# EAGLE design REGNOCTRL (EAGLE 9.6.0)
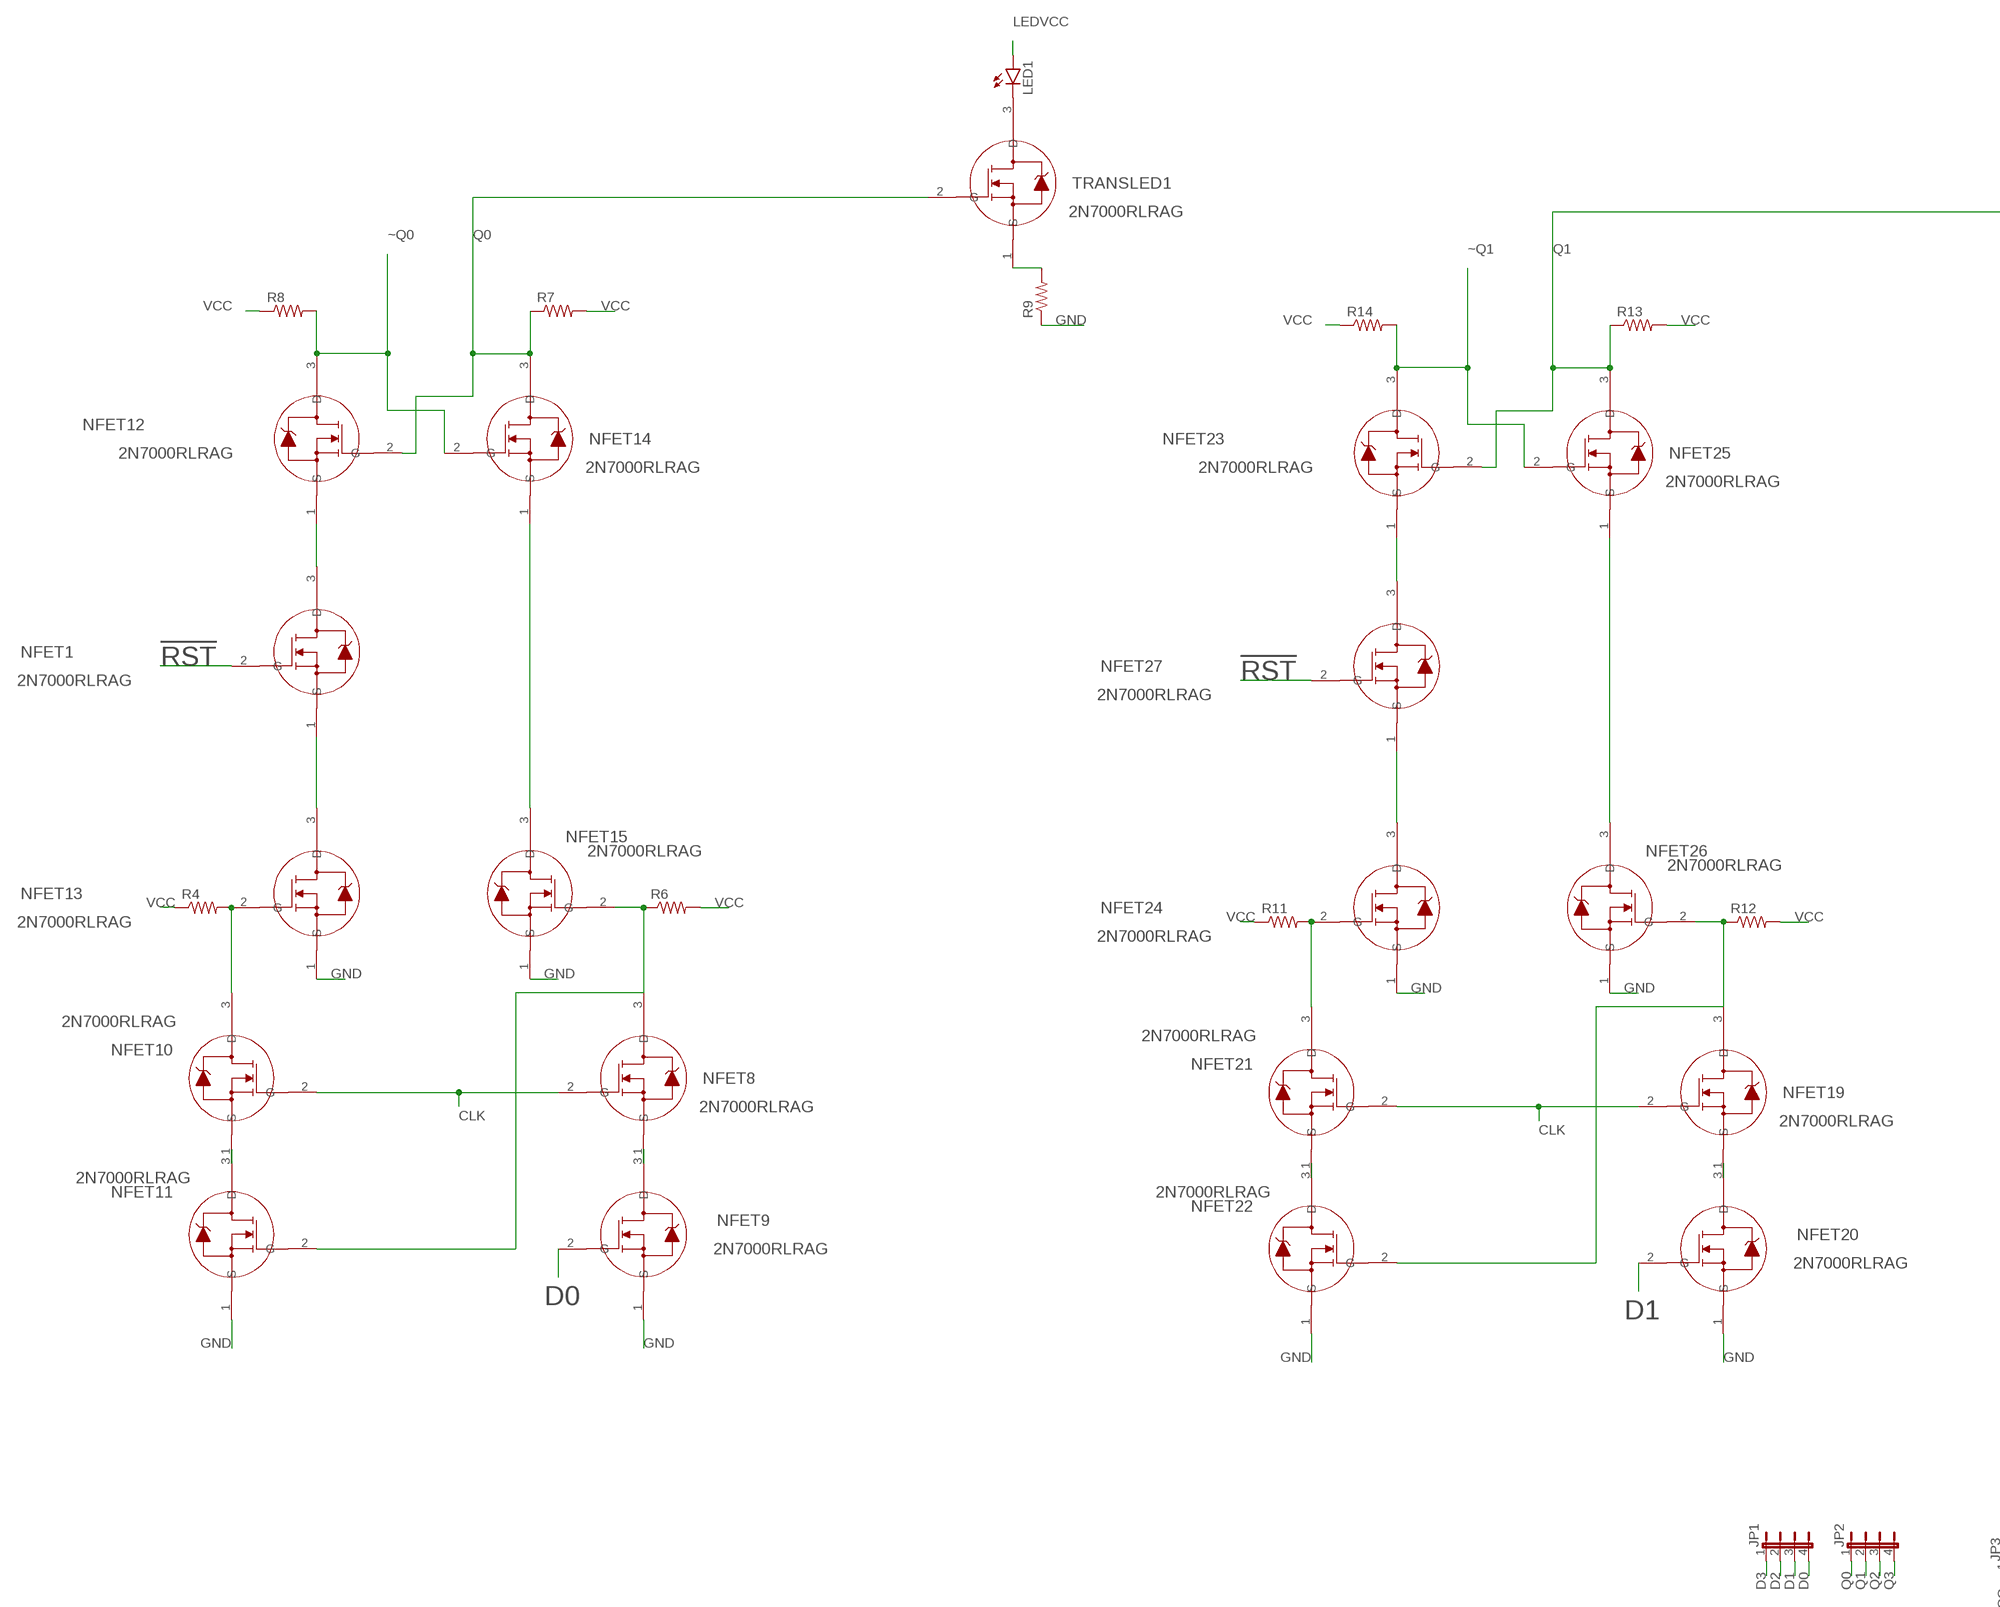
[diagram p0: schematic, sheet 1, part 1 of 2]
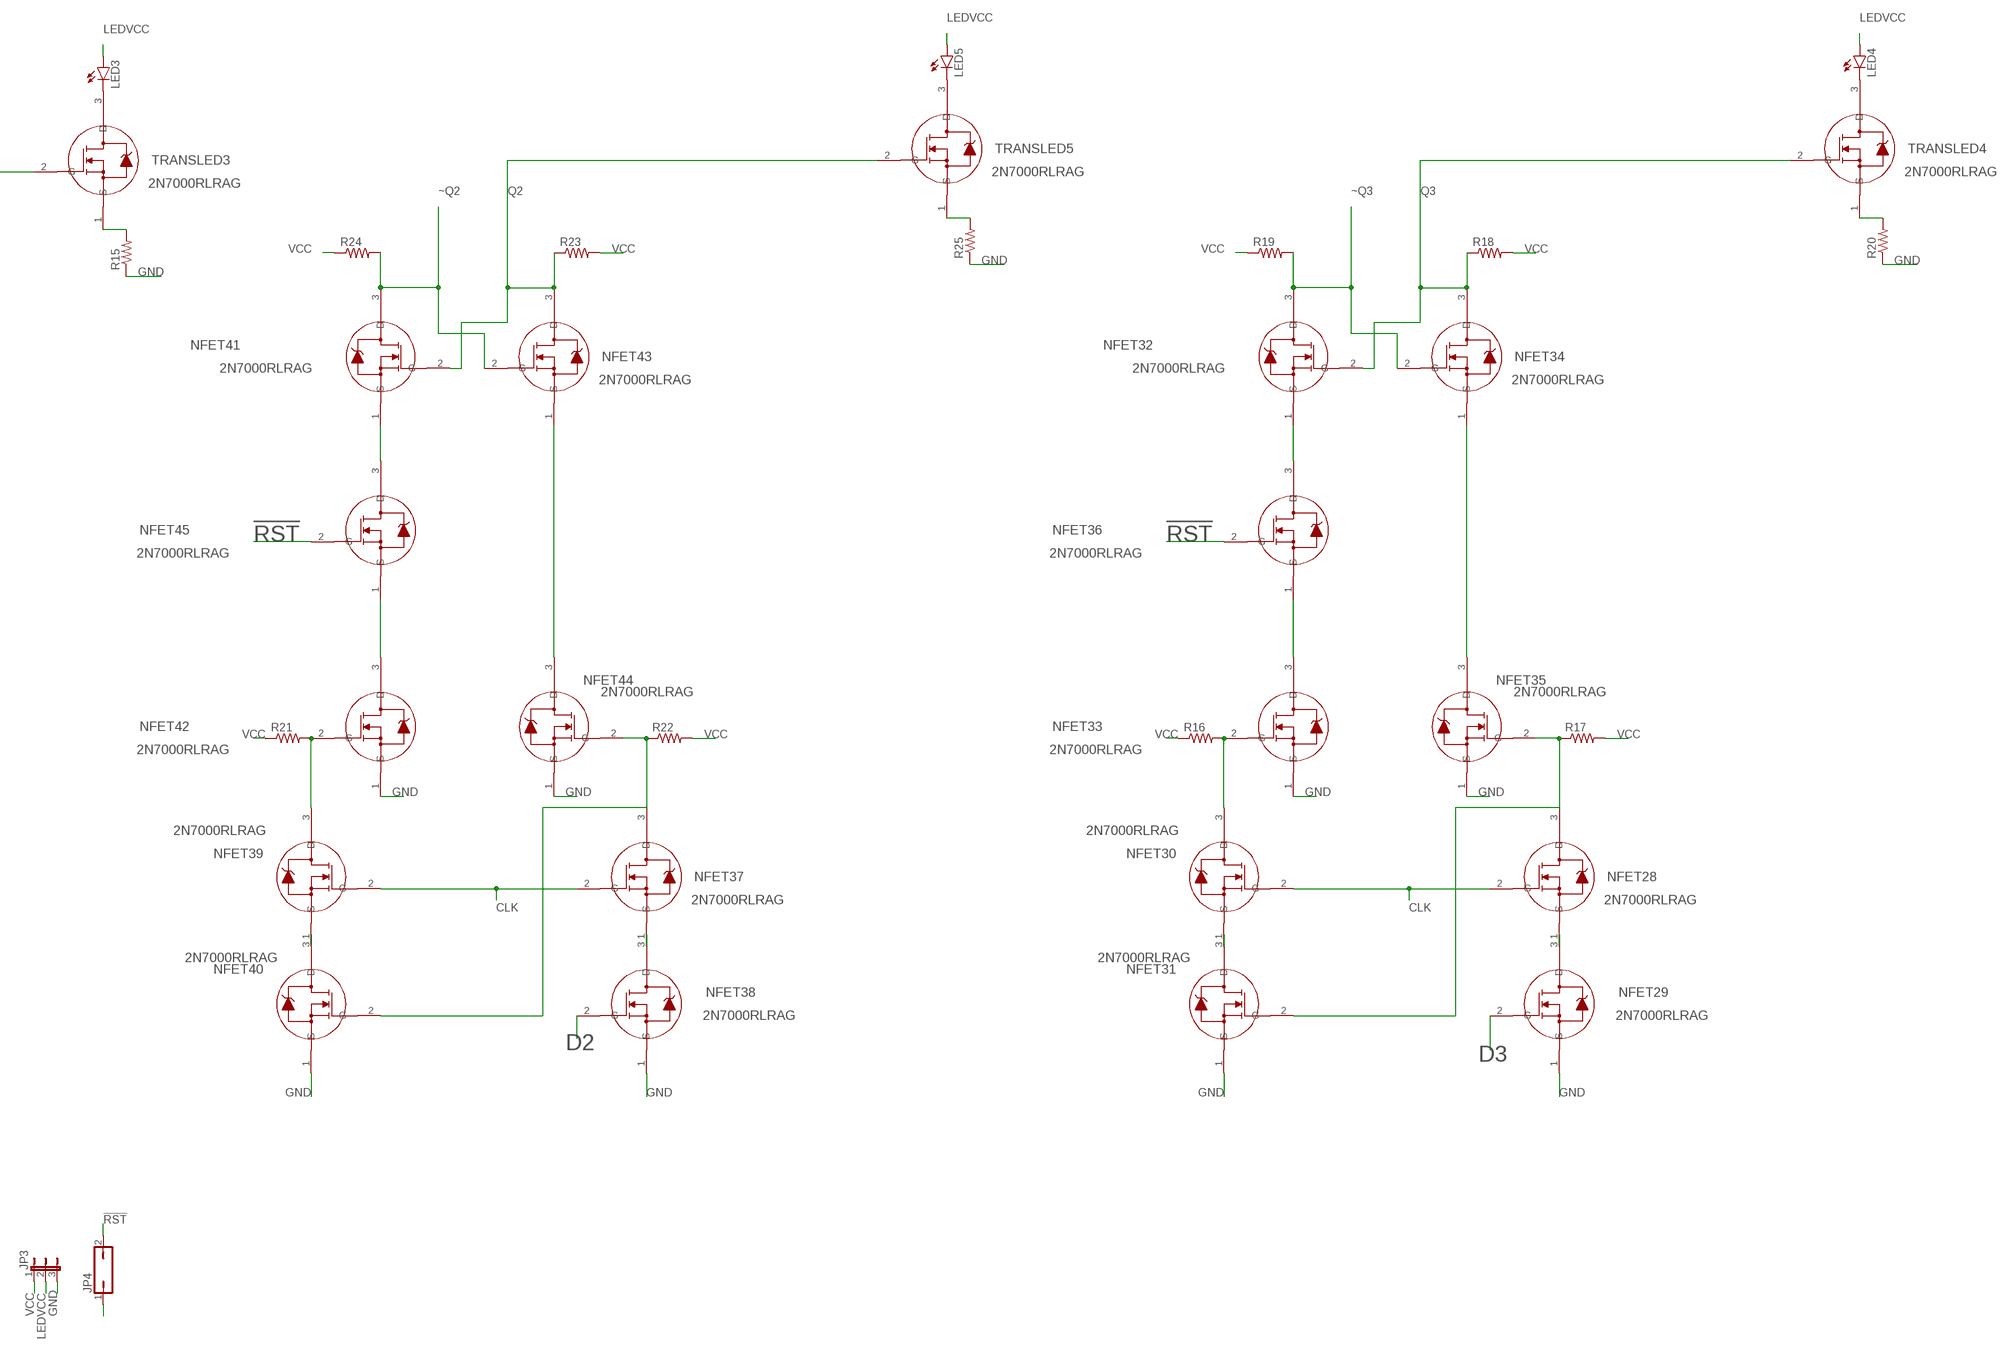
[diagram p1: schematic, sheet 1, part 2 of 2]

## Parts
JP1  JP4E  [JP4]
JP2  JP4E  [JP4]
JP3  JP2E  [JP2]
JP4  JP1Q  [JP1]
LED1  LED3MM  [LED3MM]
LED3  LED3MM  [LED3MM]
LED4  LED3MM  [LED3MM]
LED5  LED3MM  [LED3MM]
NFET1  2N7000RLRAG  [TO-92_ONS]
NFET8  2N7000RLRAG  [TO-92_ONS]
NFET9  2N7000RLRAG  [TO-92_ONS]
NFET10  2N7000RLRAG  [TO-92_ONS]
NFET11  2N7000RLRAG  [TO-92_ONS]
NFET12  2N7000RLRAG  [TO-92_ONS]
NFET13  2N7000RLRAG  [TO-92_ONS]
NFET14  2N7000RLRAG  [TO-92_ONS]
NFET15  2N7000RLRAG  [TO-92_ONS]
NFET19  2N7000RLRAG  [TO-92_ONS]
NFET20  2N7000RLRAG  [TO-92_ONS]
NFET21  2N7000RLRAG  [TO-92_ONS]
NFET22  2N7000RLRAG  [TO-92_ONS]
NFET23  2N7000RLRAG  [TO-92_ONS]
NFET24  2N7000RLRAG  [TO-92_ONS]
NFET25  2N7000RLRAG  [TO-92_ONS]
NFET26  2N7000RLRAG  [TO-92_ONS]
NFET27  2N7000RLRAG  [TO-92_ONS]
NFET28  2N7000RLRAG  [TO-92_ONS]
NFET29  2N7000RLRAG  [TO-92_ONS]
NFET30  2N7000RLRAG  [TO-92_ONS]
NFET31  2N7000RLRAG  [TO-92_ONS]
NFET32  2N7000RLRAG  [TO-92_ONS]
NFET33  2N7000RLRAG  [TO-92_ONS]
NFET34  2N7000RLRAG  [TO-92_ONS]
NFET35  2N7000RLRAG  [TO-92_ONS]
NFET36  2N7000RLRAG  [TO-92_ONS]
NFET37  2N7000RLRAG  [TO-92_ONS]
NFET38  2N7000RLRAG  [TO-92_ONS]
NFET39  2N7000RLRAG  [TO-92_ONS]
NFET40  2N7000RLRAG  [TO-92_ONS]
NFET41  2N7000RLRAG  [TO-92_ONS]
NFET42  2N7000RLRAG  [TO-92_ONS]
NFET43  2N7000RLRAG  [TO-92_ONS]
NFET44  2N7000RLRAG  [TO-92_ONS]
NFET45  2N7000RLRAG  [TO-92_ONS]
R4  R-US_0204/7  [0204/7]
R6  R-US_0204/7  [0204/7]
R7  R-US_0204/7  [0204/7]
R8  R-US_0204/7  [0204/7]
R9  R-US_0204/7  [0204/7]
R11  R-US_0204/7  [0204/7]
R12  R-US_0204/7  [0204/7]
R13  R-US_0204/7  [0204/7]
R14  R-US_0204/7  [0204/7]
R15  R-US_0204/7  [0204/7]
R16  R-US_0204/7  [0204/7]
R17  R-US_0204/7  [0204/7]
R18  R-US_0204/7  [0204/7]
R19  R-US_0204/7  [0204/7]
R20  R-US_0204/7  [0204/7]
R21  R-US_0204/7  [0204/7]
R22  R-US_0204/7  [0204/7]
R23  R-US_0204/7  [0204/7]
R24  R-US_0204/7  [0204/7]
R25  R-US_0204/7  [0204/7]
TRANSLED1  2N7000RLRAG  [TO-92_ONS]
TRANSLED3  2N7000RLRAG  [TO-92_ONS]
TRANSLED4  2N7000RLRAG  [TO-92_ONS]
TRANSLED5  2N7000RLRAG  [TO-92_ONS]

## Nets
!RST: JP4.2 NFET1.2(G) NFET27.2(G) NFET36.2(G) NFET45.2(G)
CLK: JP4.1 NFET8.2(G) NFET10.2(G) NFET19.2(G) NFET21.2(G) NFET28.2(G) NFET30.2(G) NFET37.2(G) NFET39.2(G)
D0: JP1.4 NFET9.2(G)
D1: JP1.3 NFET20.2(G)
D2: JP1.2 NFET38.2(G)
D3: JP1.1 NFET29.2(G)
GND: JP3.3 NFET9.1(S) NFET11.1(S) NFET13.1(S) NFET15.1(S) NFET20.1(S) NFET22.1(S) NFET24.1(S) NFET26.1(S) NFET29.1(S) NFET31.1(S) NFET33.1(S) NFET35.1(S) NFET38.1(S) NFET40.1(S) NFET42.1(S) NFET44.1(S) R9.1 R15.1 R20.1 R25.1
LEDVCC: JP3.2 LED1.A LED3.A LED4.A LED5.A
N$1: NFET8.1(S) NFET9.3(D)
N$2: NFET1.3(D) NFET12.1(S)
N$3: NFET10.1(S) NFET11.3(D)
N$4: NFET10.3(D) NFET13.2(G) R4.2
N$5: NFET1.1(S) NFET13.3(D)
N$6: NFET14.1(S) NFET15.3(D)
N$7: NFET8.3(D) NFET11.2(G) NFET15.2(G) R6.1
N$8: LED1.K(C) TRANSLED1.3(D)
N$10: R9.2 TRANSLED1.1(S)
N$19: NFET19.1(S) NFET20.3(D)
N$20: NFET21.1(S) NFET22.3(D)
N$21: NFET21.3(D) NFET24.2(G) R11.2
N$22: NFET25.1(S) NFET26.3(D)
N$23: NFET19.3(D) NFET22.2(G) NFET26.2(G) R12.1
N$24: LED3.K(C) TRANSLED3.3(D)
N$25: R15.2 TRANSLED3.1(S)
N$26: NFET23.1(S) NFET27.3(D)
N$27: NFET24.3(D) NFET27.1(S)
N$28: NFET28.1(S) NFET29.3(D)
N$29: NFET30.1(S) NFET31.3(D)
N$30: NFET30.3(D) NFET33.2(G) R16.2
N$31: NFET34.1(S) NFET35.3(D)
N$32: NFET28.3(D) NFET31.2(G) NFET35.2(G) R17.1
N$33: LED4.K(C) TRANSLED4.3(D)
N$34: R20.2 TRANSLED4.1(S)
N$35: NFET32.1(S) NFET36.3(D)
N$36: NFET33.3(D) NFET36.1(S)
N$37: NFET37.1(S) NFET38.3(D)
N$38: NFET39.1(S) NFET40.3(D)
N$39: NFET39.3(D) NFET42.2(G) R21.2
N$40: NFET43.1(S) NFET44.3(D)
N$41: NFET37.3(D) NFET40.2(G) NFET44.2(G) R22.1
N$42: LED5.K(C) TRANSLED5.3(D)
N$43: R25.2 TRANSLED5.1(S)
N$44: NFET41.1(S) NFET45.3(D)
N$45: NFET42.3(D) NFET45.1(S)
Q0: JP2.1 NFET12.2(G) NFET14.3(D) R7.1 TRANSLED1.2(G)
Q1: JP2.2 NFET23.2(G) NFET25.3(D) R13.1 TRANSLED3.2(G)
Q2: JP2.3 NFET41.2(G) NFET43.3(D) R23.1 TRANSLED5.2(G)
Q3: JP2.4 NFET32.2(G) NFET34.3(D) R18.1 TRANSLED4.2(G)
VCC: JP3.1 R4.1 R6.2 R7.2 R8.1 R11.1 R12.2 R13.2 R14.1 R16.1 R17.2 R18.2 R19.1 R21.1 R22.2 R23.2 R24.1
~Q0: NFET12.3(D) NFET14.2(G) R8.2
~Q1: NFET23.3(D) NFET25.2(G) R14.2
~Q2: NFET41.3(D) NFET43.2(G) R24.2
~Q3: NFET32.3(D) NFET34.2(G) R19.2

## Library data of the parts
JP1 JP2 = jumper:JP4E: JUMPER
JP3 = jumper:JP2E: JUMPER
JP4 = jumper:JP1Q: JUMPER
LED1 LED3-LED5 = led:LED: LED
NFET1 NFET8-NFET15 NFET19-NFET45 TRANSLED1 TRANSLED3-TRANSLED5 = Transistor(MOSFET):2N7000RLRAG; COPYRIGHT: Copyright (C) 2022 Ultra Librarian. All rights reserved.; MANUFACTURER_PART_NUMBER: 2N7000RLRAG; MFR_NAME: onsemi
R4 R6-R9 R11-R25 = rcl:R-US_: RESISTOR, American symbol; SPICEPREFIX: R

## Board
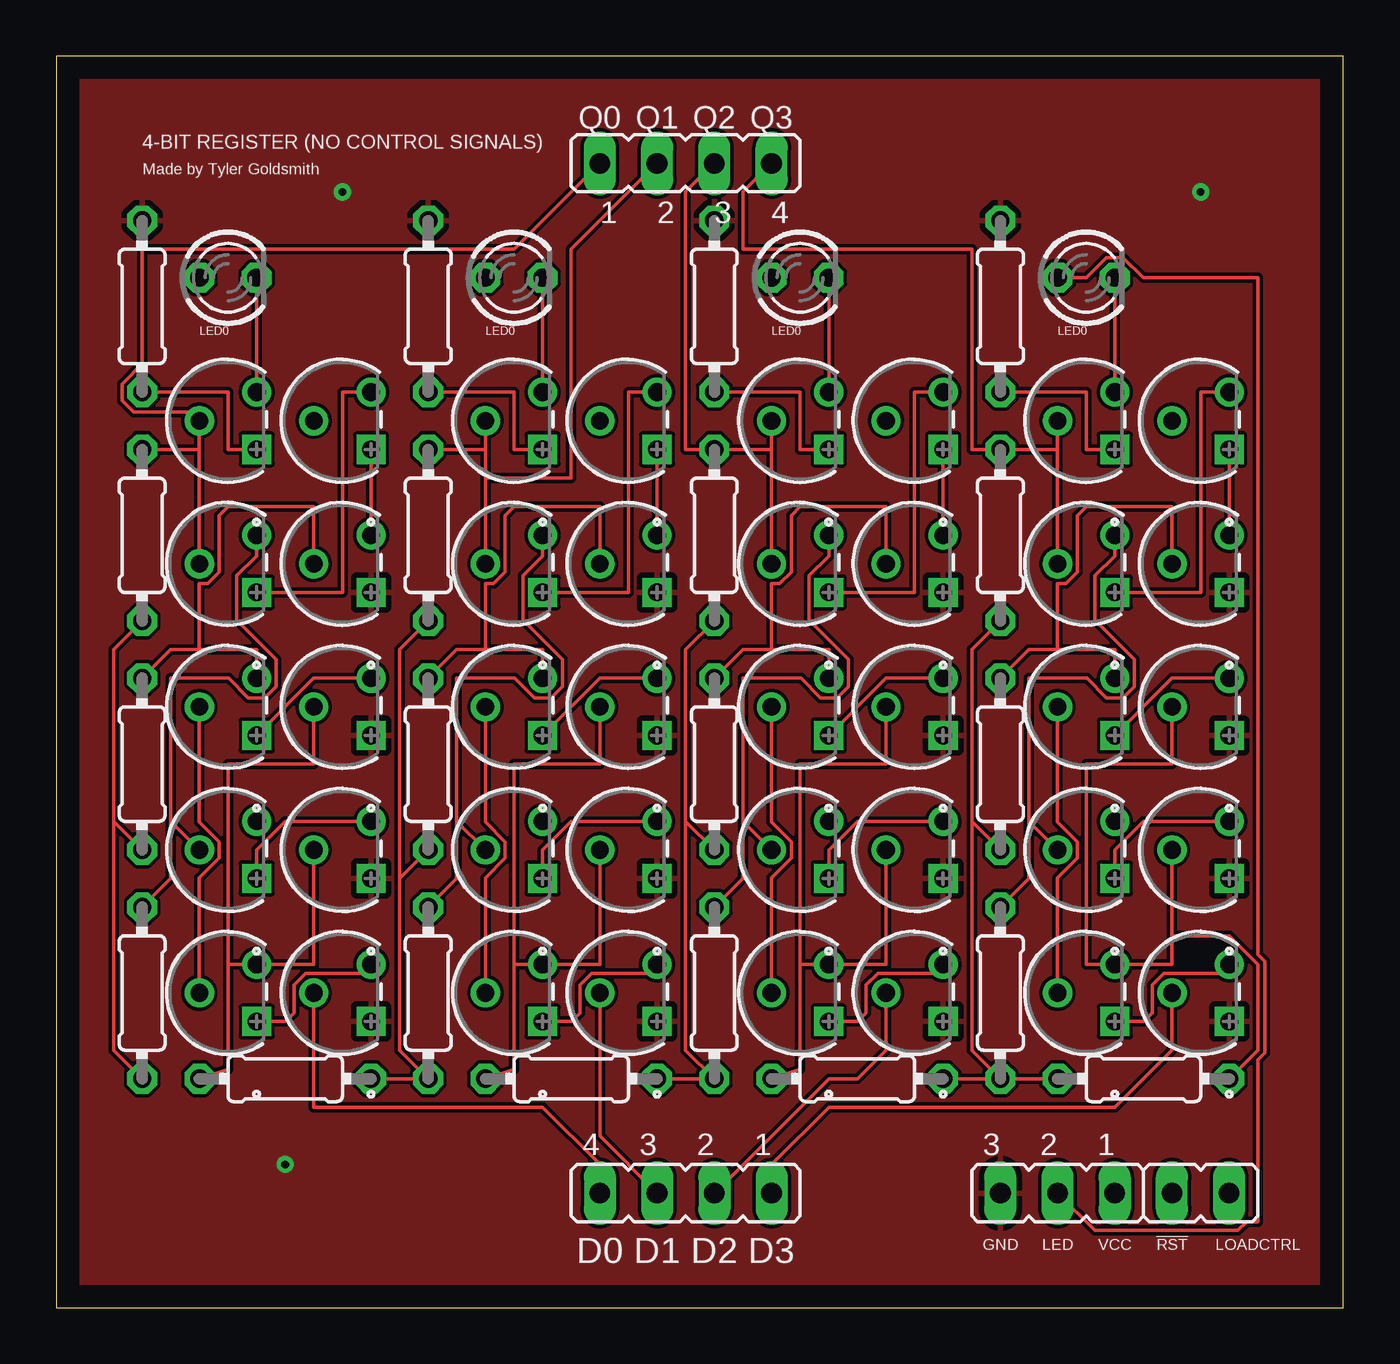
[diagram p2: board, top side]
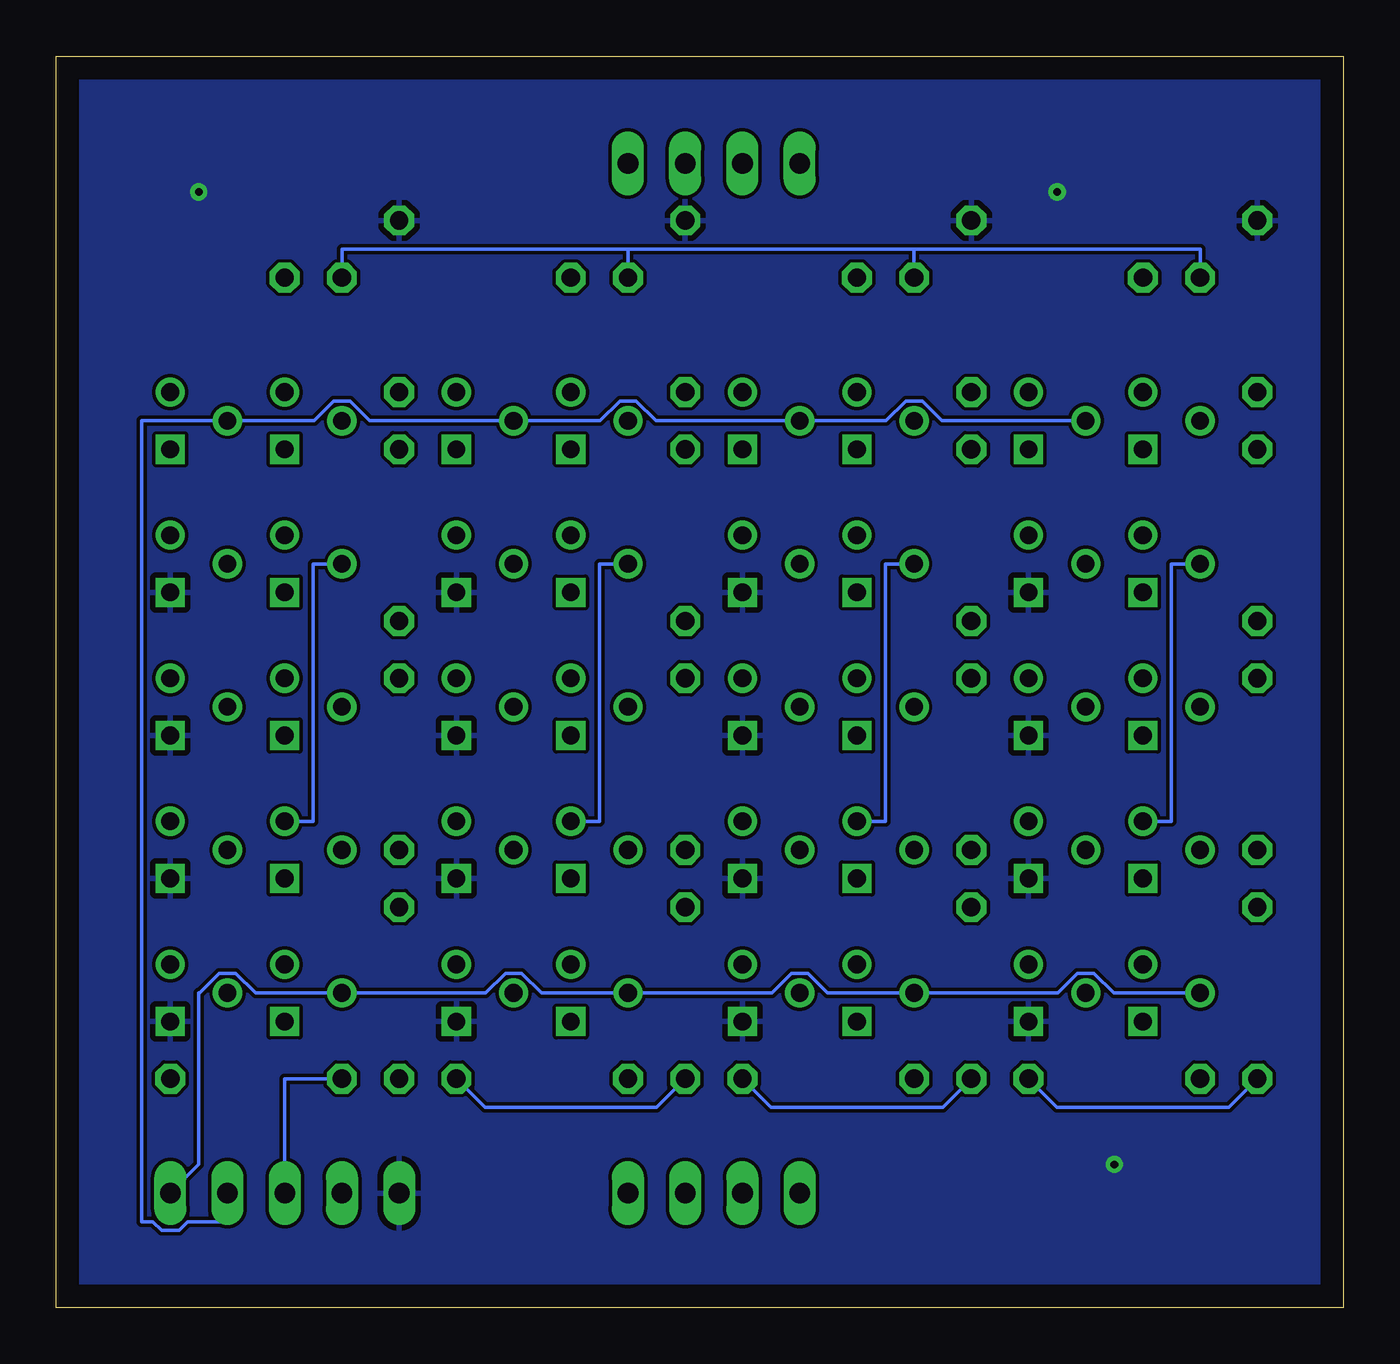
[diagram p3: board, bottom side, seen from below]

Size 57.13 x 55.55 mm. Coordinates in mm from the lower left corner, seen from the top.
Outline: 0,0 57.13,0 57.13,55.55 0,55.55 0,0
Copper layers (1*16): Top 0.035mm / dielectric 1.5mm / Bottom 0.035mm
Design rules "default": minimum track width 6mil, minimum drill 0.35mm, track to track 6mil, track to pad 6mil, pad to pad 6mil, via to via 6mil, smd to smd 6mil, copper to edge 40mil, drill to drill 6mil, minimum pad ring 10mil, minimum via ring 8mil, stop-mask expansion 4mil, vias tented up to drill 0mil, thermal gap 10mil

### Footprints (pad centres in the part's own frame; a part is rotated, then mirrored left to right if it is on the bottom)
JP4 = drill 0.914 long: 1 -3.81,0; 2 -1.27,0; 3 1.27,0; 4 3.81,0
JP2 = drill 0.914 long: 1 -2.54,0; 2 0,0; 3 2.54,0
JP1 = drill 0.914 long: 1 0,-1.27; 2 0,1.27
LED3MM = drill 0.813 octagon: A -1.27,0; K 1.27,0
TO-92_ONS = drill 0.787 pad 1.295 square: 1 0,0 | drill 0.787 pad 1.295: 2 1.27,2.54; 3 2.54,0
0204/7 = drill 0.813 octagon: 1 -3.81,0; 2 3.81,0

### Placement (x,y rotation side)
JP1  27.94,5.08 180 top
JP2  27.94,50.8 0 top
JP3  44.45,5.08 180 top
JP4  50.8,5.08 90 top
LED1  7.62,45.72 0 top
LED3  20.32,45.72 0 top
LED4  45.72,45.72 0 top
LED5  33.02,45.72 0 top
NFET1  13.97,38.1 90 top
NFET8  8.89,12.7 90 top
NFET9  13.97,12.7 90 top
NFET10  8.89,25.4 90 top
NFET11  13.97,25.4 90 top
NFET12  8.89,31.75 90 top
NFET13  13.97,31.75 90 top
NFET14  8.89,19.05 90 top
NFET15  13.97,19.05 90 top
NFET19  21.59,12.7 90 top
NFET20  26.67,12.7 90 top
NFET21  21.59,25.4 90 top
NFET22  26.67,25.4 90 top
NFET23  21.59,31.75 90 top
NFET24  26.67,31.75 90 top
NFET25  21.59,19.05 90 top
NFET26  26.67,19.05 90 top
NFET27  26.67,38.1 90 top
NFET28  46.99,12.7 90 top
NFET29  52.07,12.7 90 top
NFET30  46.99,25.4 90 top
NFET31  52.07,25.4 90 top
NFET32  46.99,31.75 90 top
NFET33  52.07,31.75 90 top
NFET34  46.99,19.05 90 top
NFET35  52.07,19.05 90 top
NFET36  52.07,38.1 90 top
NFET37  34.29,12.7 90 top
NFET38  39.37,12.7 90 top
NFET39  34.29,25.4 90 top
NFET40  39.37,25.4 90 top
NFET41  34.29,31.75 90 top
NFET42  39.37,31.75 90 top
NFET43  34.29,19.05 90 top
NFET44  39.37,19.05 90 top
NFET45  39.37,38.1 90 top
R4  3.81,24.13 90 top
R6  10.16,10.16 0 top
R7  3.81,34.29 270 top
R8  3.81,13.97 90 top
R9  3.81,44.45 270 top
R11  16.51,24.13 90 top
R12  22.86,10.16 0 top
R13  16.51,34.29 270 top
R14  16.51,13.97 90 top
R15  16.51,44.45 270 top
R16  41.91,24.13 90 top
R17  48.26,10.16 180 top
R18  41.91,34.29 270 top
R19  41.91,13.97 90 top
R20  41.91,44.45 270 top
R21  29.21,24.13 90 top
R22  35.56,10.16 0 top
R23  29.21,34.29 270 top
R24  29.21,13.97 90 top
R25  29.21,44.45 270 top
TRANSLED1  8.89,38.1 90 top
TRANSLED3  21.59,38.1 90 top
TRANSLED4  46.99,38.1 90 top
TRANSLED5  34.29,38.1 90 top

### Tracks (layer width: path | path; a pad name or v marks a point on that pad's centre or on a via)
!RST
  Bottom 0.152: NFET1.2 17.81,39.37 18.69,40.25 19.41,40.25 20.29,39.37 NFET27.2 30.51,39.37 31.39,40.25 32.11,40.25 32.99,39.37 NFET45.2 43.21,39.37 44.09,40.25 44.81,40.25 45.69,39.37 NFET36.2 53.34,39.37 53.34,3.81 52.84,3.81 52.46,3.43 51.68,3.43 51.3,3.81 49.53,3.81 JP4.2
CLK
  Top 0.152: NFET10.2 6.35,21.56 7.23,20.68 7.23,19.96 6.35,19.08 NFET8.2 | NFET21.2 19.05,21.56 19.93,20.68 19.93,19.96 19.05,19.08 NFET19.2 | NFET39.2 31.75,21.56 32.63,20.68 32.63,19.96 31.75,19.08 NFET37.2 | NFET30.2 44.45,21.56 45.33,20.68 45.33,19.96 44.45,19.08 NFET28.2
  Bottom 0.152: NFET8.2 10.19,13.97 11.07,14.85 11.79,14.85 12.67,13.97 NFET19.2 22.89,13.97 23.77,14.85 24.49,14.85 25.37,13.97 NFET37.2 35.59,13.97 36.47,14.85 37.19,14.85 38.07,13.97 NFET28.2 48.29,13.97 49.17,14.85 49.89,14.85 50.77,13.97 50.8,13.97 50.8,6.35 JP4.1
D0
  Top 0.152: NFET9.2 11.43,8.89 21.59,8.89 24.13,6.35 JP1.4
D1
  Top 0.152: JP1.3 24.13,7.62 NFET20.2
D2
  Top 0.152: NFET38.2 36.83,11.43 35.56,10.16 34.29,10.16 JP1.2
D3
  Top 0.152: JP1.1 31.75,6.35 34.29,8.89 46.99,8.89 49.53,11.43 NFET29.2
GND  (via drill 0.35)
  other vias: 50.8,49.53 10.16,6.35 12.7,49.53
  pour Top: -1.27,55.88 57.15,55.88 57.15,0 0,0 0,54.61
  pour Bottom: -1.27,55.88 57.15,55.88 57.15,0 0,0 0,54.61
LEDVCC
  Top 0.152: JP3.2 46.1,3.43 52.46,3.43 52.84,3.81 53.34,3.81 53.34,11 53.65,11.3 53.65,15.37 53.34,15.67 53.34,45.72 48.25,45.72 47.36,46.61 46.62,46.61 45.73,45.72 LED4.A
  Bottom 0.152: LED5.A 31.75,46.99 | 31.75,46.99 44.45,46.99 LED4.A | 31.75,46.99 19.05,46.99 | 19.05,46.99 LED3.A | LED1.A 6.35,46.99 19.05,46.99
N$1
  Top 0.152: NFET8.1 10.16,12.7 10.55,13.09 10.55,14.33 11.07,14.85 13.58,14.85 NFET9.3
N$2
  Top 0.152: NFET12.1 12.7,31.75 12.7,40.64 NFET1.3
N$3
  Top 0.152: NFET10.1 11.43,27.94 NFET11.3
N$4
  Top 0.152: NFET10.3 8.89,29.21 6.35,29.21 | NFET13.2 11.43,35.56 7.62,35.56 7.23,35.17 7.23,32.66 6.71,32.14 6.35,32.14 6.35,29.21 | R4.2 5.08,29.21 6.35,29.21
N$5
  Top 0.152: NFET13.3 NFET1.1
N$6
  Top 0.152: NFET15.3 10.16,21.59 8.89,20.32 NFET14.1
N$7
  Top 0.152: NFET15.2 11.43,15.24 NFET8.3 7.62,15.24 | 7.62,15.24 7.62,10.58 R6.1 | 7.62,15.24 7.62,24.13 11.43,24.13 NFET11.2
N$8
  Top 0.152: TRANSLED1.3 LED1.K
N$10
  Top 0.152: TRANSLED1.1 7.62,38.1 7.62,40.64 R9.2
N$19
  Top 0.152: NFET19.1 22.86,12.7 23.25,13.09 23.25,14.33 23.77,14.85 26.28,14.85 NFET20.3
N$20
  Top 0.152: NFET21.1 24.13,27.94 NFET22.3
N$21
  Top 0.152: NFET21.3 21.59,29.21 19.05,29.21 | NFET24.2 24.13,35.56 20.32,35.56 19.93,35.17 19.93,32.66 19.41,32.14 19.05,32.14 19.05,29.21 | R11.2 17.78,29.21 19.05,29.21
N$22
  Top 0.152: NFET26.3 22.86,21.59 21.59,20.32 NFET25.1
N$23
  Top 0.152: NFET26.2 24.13,15.24 NFET19.3 20.32,15.24 | 20.32,15.24 20.32,10.58 R12.1 | 20.32,15.24 20.32,24.13 24.13,24.13 NFET22.2
N$24
  Top 0.152: TRANSLED3.3 LED3.K
N$25
  Top 0.152: TRANSLED3.1 20.32,38.1 20.32,40.64 R15.2
N$26
  Top 0.152: NFET23.1 25.4,31.75 25.4,40.64 NFET27.3
N$27
  Top 0.152: NFET24.3 NFET27.1
N$28
  Top 0.152: NFET28.1 48.26,12.7 48.65,13.09 48.65,14.33 49.17,14.85 51.68,14.85 NFET29.3
N$29
  Top 0.152: NFET30.1 49.53,27.94 NFET31.3
N$30
  Top 0.152: NFET30.3 46.99,29.21 44.45,29.21 | NFET33.2 49.53,35.56 45.72,35.56 45.33,35.17 45.33,32.66 44.81,32.14 44.45,32.14 44.45,29.21 | R16.2 43.18,29.21 44.45,29.21
N$31
  Top 0.152: NFET35.3 48.26,21.59 46.99,20.32 NFET34.1
N$32
  Top 0.152: NFET35.2 49.53,16.51 | 49.53,16.51 49.53,15.24 NFET28.3 45.72,15.24 45.72,24.13 49.53,24.13 NFET31.2 | R17.1 53.34,11.43 53.34,15.24 52.07,16.51 49.53,16.51
N$33
  Top 0.152: TRANSLED4.3 LED4.K
N$34
  Top 0.152: TRANSLED4.1 45.72,38.1 45.72,40.64 R20.2
N$35
  Top 0.152: NFET32.1 50.8,31.75 50.8,40.64 NFET36.3
N$36
  Top 0.152: NFET33.3 NFET36.1
N$37
  Top 0.152: NFET37.1 35.56,12.7 35.95,13.09 35.95,14.33 36.47,14.85 38.98,14.85 NFET38.3
N$38
  Top 0.152: NFET39.1 36.83,27.94 NFET40.3
N$39
  Top 0.152: NFET39.3 34.29,29.21 31.75,29.21 | NFET42.2 36.83,35.56 33.02,35.56 32.63,35.17 32.63,32.66 32.11,32.14 31.75,32.14 31.75,29.21 | R21.2 30.48,29.21 31.75,29.21
N$40
  Top 0.152: NFET44.3 35.56,21.59 34.29,20.32 NFET43.1
N$41
  Top 0.152: NFET44.2 36.83,15.24 NFET37.3 33.02,15.24 | 33.02,15.24 33.02,10.58 R22.1 | 33.02,15.24 33.02,24.13 36.83,24.13 NFET40.2
N$42
  Top 0.152: TRANSLED5.3 LED5.K
N$43
  Top 0.152: TRANSLED5.1 33.02,38.1 33.02,40.64 R25.2
N$44
  Top 0.152: NFET41.1 38.1,31.75 38.1,40.64 NFET45.3
N$45
  Top 0.152: NFET42.3 NFET45.1
Q0
  Top 0.152: NFET12.2 6.35,38.1 | 6.35,38.1 TRANSLED1.2 5.97,39.75 3.44,39.75 2.92,40.27 2.92,41.01 3.81,41.9 3.81,46.99 20.32,46.99 JP2.1 | R7.1 6.35,38.1
  Bottom 0.152: NFET12.2 7.62,33.02 7.62,21.59 NFET14.3
Q1
  Top 0.152: NFET23.2 19.05,36.83 | 19.05,36.83 19.05,38.1 | 19.05,38.1 TRANSLED3.2 | R13.1 19.05,38.1 | 19.05,36.83 22.86,36.83 22.86,46.99 JP2.2
  Bottom 0.152: NFET23.2 20.32,33.02 20.32,21.59 NFET25.3
Q2
  Top 0.152: NFET41.2 31.75,38.1 | 31.75,38.1 TRANSLED5.2 | 31.75,38.1 R23.1 27.94,38.1 27.94,49.53 JP2.3
  Bottom 0.152: NFET41.2 33.02,33.02 33.02,21.59 NFET43.3
Q3
  Top 0.152: NFET32.2 44.45,38.1 | 44.45,38.1 TRANSLED4.2 | 44.45,38.1 R18.1 40.64,38.1 40.64,46.99 30.48,46.99 30.48,49.53 JP2.4
  Bottom 0.152: NFET32.2 45.72,33.02 45.72,21.59 NFET34.3
VCC
  Top 0.152: R4.1 2.54,21.59 | 2.54,21.59 2.54,29.21 R7.2 | R8.1 2.54,11.43 2.54,21.59 | 15.24,19.05 15.24,11.43 R14.1 R6.2 | R11.1 15.24,19.05 | 15.24,19.05 15.24,29.21 R13.2 | R23.2 27.94,29.21 27.94,21.59 | 27.94,21.59 R21.1 | 27.94,21.59 27.94,11.43 R24.1 R12.2 | R22.2 R19.1 | R17.2 R19.1 | R16.1 40.64,21.59 | 40.64,21.59 40.64,29.21 R18.2 | R19.1 40.64,11.43 40.64,21.59
  Bottom 0.152: JP3.1 46.99,10.16 R17.2 | R8.1 5.08,8.89 12.7,8.89 R6.2 | R14.1 17.78,8.89 25.4,8.89 R12.2 | R24.1 30.48,8.89 38.1,8.89 R22.2
~Q0
  Top 0.152: NFET14.2 5.08,21.59 | 5.08,21.59 5.08,27.94 7.65,27.94 8.53,27.06 9.25,27.06 9.77,27.58 9.77,28.77 8.01,30.52 8.01,32.49 8.89,33.37 NFET12.3 | R8.2 5.08,19.05 5.08,21.59
~Q1
  Top 0.152: NFET25.2 17.78,21.59 | 17.78,21.59 17.78,27.94 20.35,27.94 21.23,27.06 21.95,27.06 22.47,27.58 22.47,28.77 20.71,30.52 20.71,32.49 21.59,33.37 NFET23.3 | R14.2 17.78,19.05 17.78,21.59
~Q2
  Top 0.152: NFET43.2 30.48,21.59 | 30.48,21.59 30.48,27.94 33.05,27.94 33.93,27.06 34.65,27.06 35.17,27.58 35.17,28.77 33.41,30.52 33.41,32.49 34.29,33.37 NFET41.3 | R24.2 30.48,19.05 30.48,21.59
~Q3
  Top 0.152: NFET34.2 43.18,21.59 | 43.18,21.59 43.18,27.94 45.75,27.94 46.63,27.06 47.35,27.06 47.87,27.58 47.87,28.77 46.11,30.52 46.11,32.49 46.99,33.37 NFET32.3 | R19.2 43.18,19.05 43.18,21.59

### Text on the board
tNames: Q0 | Q1 | Q2 | Q3 | 4-BIT REGISTER (NO CONTROL SIGNALS) | Made by Tyler Goldsmith | LED0 | LED0 | LED0 | LED0 | D0 | D1 | D2 | D3 | GND | LED | VCC | !RST | LOADCTRL | LOADCTRL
